INTERFACE ICylinder

METHOD M_MoveToBase : BOOL
VAR_INPUT
END_VAR
END_METHOD

METHOD M_MoveToWork : BOOL
VAR_INPUT
END_VAR
END_METHOD

METHOD M_Reset
VAR_INPUT
END_VAR
END_METHOD

METHOD M_StateMachine : BOOL
VAR_INPUT
	bBasePosReq		: BOOL;
	bWorkPosReq		: BOOL;
END_VAR
END_METHOD

PROPERTY P_AtBasePos : BOOL
GET
END_GET
SET
END_SET
END_PROPERTY

PROPERTY P_AtWorkPos : BOOL
GET
END_GET
SET
END_SET
END_PROPERTY

PROPERTY P_ToWork : BOOL
GET
END_GET
SET
END_SET
END_PROPERTY

END_INTERFACE
